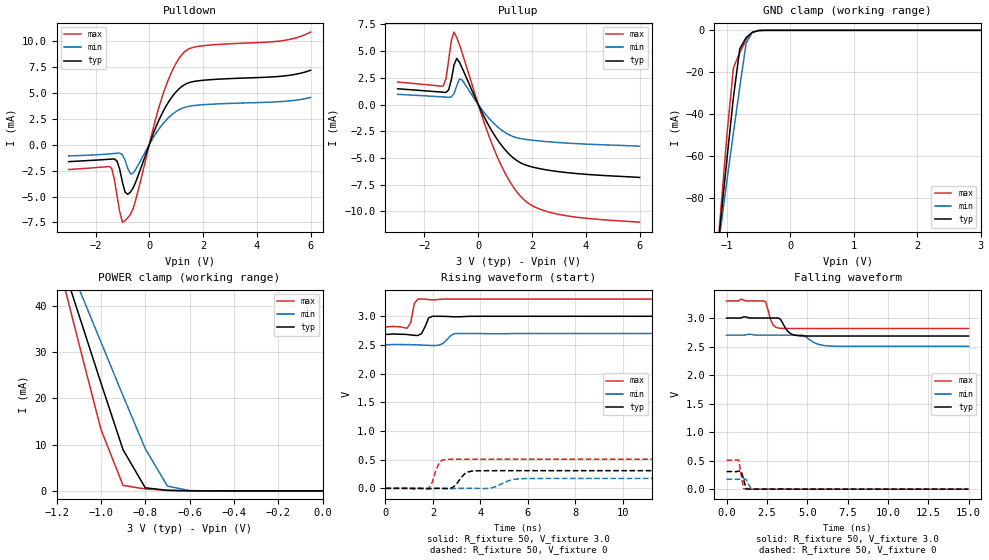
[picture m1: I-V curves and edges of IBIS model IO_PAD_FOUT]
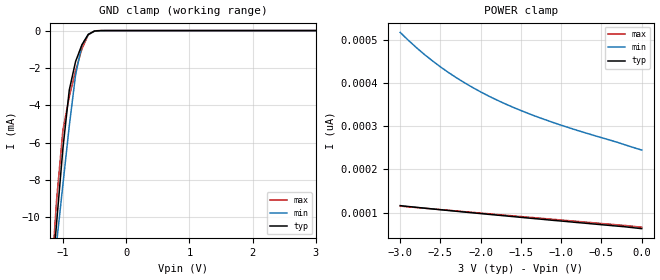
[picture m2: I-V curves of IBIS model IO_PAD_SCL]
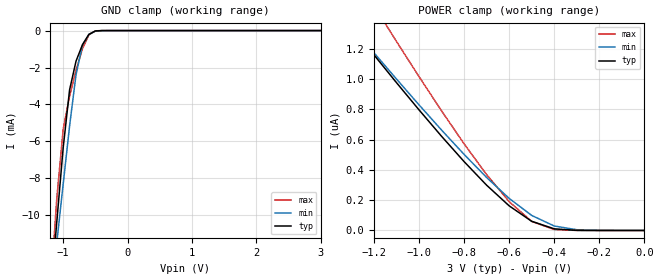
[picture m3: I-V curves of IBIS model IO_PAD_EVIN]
[IBIS Ver]   3.2
[Comment Char]   |_char
[File name]   rx8111ce_3v.ibs
[File Rev]   1.0
[Date]   2019/09/25 8:10:22
[Source]
[Notes]
[Disclaimer]
This information is for modeling purposes only, and is not guaranteed.
Property of SEIKO EPSON Corp.,
unauthorized reproduction and/or distribution is strictly prohibited.
[Copyright]
Copyright 2019, SEIKO EPSON Corp.
[Component]   T5462W0B
Si_location Pin
Timing_location Pin
[Manufacturer]   SEIKO EPSON Corp.
| RX-8111CE
[Package]
R_pkg   0.0m   0.0m   0.0m
L_pkg   0.0n   0.0n   0.0n
C_pkg   0.0p   0.0p   0.0p
[Pin] signal_name   model_name
1   VDD   POWER
2   VOUT   POWER
3   VBAT   POWER
4   FOUT   IO_PAD_FOUT
5   SCL   IO_PAD_SCL
6   EVIN   IO_PAD_EVIN
7   SDA   IO_PAD_SDA
8   VIO   POWER
9   GND   GND
10   /INT   IO_PAD_XINT
| Models and submodels in the file (5): IO_PAD_FOUT (3-state), IO_PAD_SCL (Input), IO_PAD_EVIN (Input), IO_PAD_SDA (I/O_open_drain), IO_PAD_XINT (Open_drain)
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[Model]   IO_PAD_FOUT
Model_type 3-state
Enable Active-High
Polarity Non-Inverting
Vmeas=1.50
C_comp   2.5p   2.0p   3.0p
[Temperature Range] 25   105   -40
[Voltage Range]   3.0   2.7   3.3
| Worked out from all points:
|   slope of the pulldown table from 0 to 0.45 V, typ, clamps not added: 158 ohm
|   slope of the pullup table from 0 to 0.45 V, typ, clamps not added: 202 ohm
|   GND clamp passes 1 mA (typ) near -0.60 V on its own axis
|   POWER clamp passes 1 mA (typ) near -0.80 V on its own axis
|   falling waveform, R_fixture 50, V_fixture 3.0: 20-80 % time 453ps typ, 696ps min, 319ps max; typ from 3 V to 2.69 V
|   falling waveform, R_fixture 50, V_fixture 0: 20-80 % time 184ps typ, 208ps min, 185ps max; typ from 0.309 V to 0 V
|   rising waveform, R_fixture 50, V_fixture 3.0: 20-80 % time 205ps typ, 279ps min, 132ps max; typ from 2.69 V to 3 V
|   rising waveform, R_fixture 50, V_fixture 0: 20-80 % time 365ps typ, 571ps min, 257ps max; typ from 0 V to 0.309 V
[Pullup]
-3V       1.471mA    952.6uA    2.104mA
-1.3V     1.147mA    709.8uA    1.738mA
-1.2V     1.13mA     694.5uA    2.414mA
-1.1V     1.366mA    679uA      4.16mA
-1V       2.339mA    705.4uA    6.008mA
-900mV    3.706mA    1.017mA    6.776mA
-800mV    4.313mA    1.748mA    6.271mA
-600mV    3.419mA    2.299mA    4.848mA
600mV     -2.854mA   -1.818mA   -4.245mA
1.6V      -5.487mA   -3.2mA     -8.66mA
2.9V      -6.251mA   -3.543mA   -10.23mA
6V        -6.823mA   -3.898mA   -11.01mA
[Pulldown]
-3V       -1.645mA   -1.105mA   -2.404mA
-1.4V     -1.401mA   -881.9uA   -2.281mA
-1.2V     -1.594mA   -838.2uA   -4.933mA
-1V       -3.61mA    -971.9uA   -7.472mA
-800mV    -4.793mA   -2.307mA   -7.046mA
-600mV    -4.172mA   -2.75mA    -6.158mA
500mV     3.112mA    1.977mA    4.757mA
900mV     4.773mA    3.003mA    7.349mA
1.3V      5.744mA    3.563mA    8.902mA
2V        6.182mA    3.832mA    9.508mA
5V        6.596mA    4.15mA     10.01mA
6V        7.149mA    4.527mA    10.82mA
[GND Clamp]
-3V       -666mA     -547.8mA   -822.2mA
-1.2V     -119.6mA   -117.1mA   -123.7mA
-1.1V     -89.89mA   -93.83mA   -85.8mA
-1V       -60.42mA   -70.86mA   -48.73mA
-900mV    -31.79mA   -48.51mA   -17.79mA
-800mV    -8.762mA   -26.99mA   -10.57mA
-700mV    -3.482mA   -6.087mA   -4.558mA
-600mV    -875.1uA   -938.3uA   -964.6uA
-500mV    -86.79uA   -136.7uA   -53.06uA
-400mV    -4.756uA   -14.79uA   -1.084uA
3V        37.81pA    65.05nA    23.86pA
[POWER Clamp]
-3V       323.7mA    269.5mA    395.6mA
-1.2V     53.06mA    55.67mA    50.96mA
-1.1V     38.19mA    43.92mA    32.03mA
-1V       23.39mA    32.21mA    13.33mA
-900mV    8.898mA    20.56mA    1.192mA
-800mV    679.8uA    9.149mA    426.2uA
-700mV    116.6uA    1.034mA    140.4uA
-600mV    22.63uA    76.12uA    22.74uA
0V        37.92pA    763.7pA    29.64pA
[Falling Waveform]
R_fixture=50
V_fixture=3.0
V_fixture_min=2.7
V_fixture_max=3.3
0s        3V         2.7V       3.3V
909.1ps   3.003V     2.699V     3.333V
2.424ns   3V         2.7V       3.286V
2.727ns   3V         2.7V       2.971V
2.879ns   3V         2.7V       2.883V
3.333ns   2.982V     2.7V       2.82V
3.788ns   2.77V      2.7V       2.817V
4.394ns   2.692V     2.7V       2.817V
6.364ns   2.685V     2.511V     2.816V
15ns      2.685V     2.505V     2.816V
[Falling Waveform]
R_fixture=50
V_fixture=0
V_fixture_min=0
V_fixture_max=0
0s        308.8mV    173.5mV    508.3mV
606.1ps   306.9mV    172.2mV    509.2mV
757.6ps   317.4mV    172.5mV    510.2mV
909.1ps   318.5mV    177.7mV    238.4mV
1.061ns   167.4mV    186mV      11.86mV
1.212ns   14.15mV    167.8mV    329.8uV
1.364ns   1.997mV    84.14mV    10.39uV
1.515ns   201.5uV    15.32mV    -15.29uV
1.818ns   11.09uV    1.012mV    -15.97uV
15ns      0V         0V         621.2nV
[Rising Waveform]
R_fixture=50
V_fixture=3.0
V_fixture_min=2.7
V_fixture_max=3.3
0s        2.685V     2.505V     2.816V
909.1ps   2.683V     2.506V     2.791V
1.061ns   2.675V     2.505V     2.887V
1.212ns   2.668V     2.505V     3.221V
1.364ns   2.666V     2.502V     3.299V
1.515ns   2.697V     2.499V     3.299V
1.818ns   2.971V     2.493V     3.291V
1.97ns    3V         2.491V     3.285V
3.03ns    2.991V     2.7V       3.3V
15ns      3V         2.7V       3.3V
[Rising Waveform]
R_fixture=50
V_fixture=0
V_fixture_min=0
V_fixture_max=0
0s        0V         0V         0V
1.818ns   -8.601mV   102.5uV    633.1uV
2.273ns   -361.6uV   -684.4uV   455.5mV
2.576ns   -2.263mV   -3.519mV   505.4mV
2.879ns   27.32mV    -4.664mV   507.4mV
3.333ns   253.3mV    3.654uV    508.1mV
3.788ns   305.3mV    -550.9uV   508.3mV
4.394ns   308.2mV    1.863mV    508.3mV
5.758ns   308.8mV    169.3mV    508.3mV
15ns      308.8mV    173.5mV    508.3mV
[Ramp]
R_load=50
dV/dt_r   1.853E-1/3.478E-10   1.041E-1/5.635E-10   3.050E-1/2.294E-10
dV/dt_f   1.891E-1/4.362E-10   1.172E-1/6.888E-10   2.901E-1/2.838E-10
|[End   IO_PAD_FOUT
[Model]   IO_PAD_SCL
Model_type Input
Enable Active-High
Polarity Non-Inverting
Vinh=2.64
Vinl=0.54
C_comp   2.5p   2.0p   3.0p
[Temperature Range] 25   105   -40
[Voltage Range]   3.0   2.7   3.3
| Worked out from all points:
|   GND clamp passes 1 mA (typ) near -0.73 V on its own axis
[GND Clamp]
-3V       -89.07mA   -73.01mA   -108.2mA
-1.2V     -14.34mA   -14.53mA   -14.15mA
-1.1V     -10.29mA   -11.38mA   -9.068mA
-1V       -6.299mA   -8.232mA   -5.325mA
-900mV    -3.19mA    -5.115mA   -3.551mA
-800mV    -1.656mA   -2.369mA   -2.158mA
-700mV    -763.9uA   -781.8uA   -983.1uA
-600mV    -207.7uA   -205.1uA   -228.8uA
-500mV    -21.87uA   -34.9uA    -13.49uA
-300mV    -47nA      -341.4nA   -3.543nA
3V        62.74pA    262.6pA    59.91pA
[POWER Clamp]
-3V       116.1pA    517.3pA    114.9pA
-2.9V     114.1pA    499.3pA    113.4pA
-2.7V     110.2pA    466.4pA    110.1pA
-2.5V     106.6pA    437.5pA    106.9pA
-2.2V     101.2pA    400.6pA    102pA
-1.9V     95.86pA    369.8pA    97.27pA
-1.6V     90.66pA    344.1pA    92.38pA
-1.2V     83.74pA    315.2pA    85.98pA
-800mV    76.94pA    290.4pA    79.61pA
0V        62.73pA    244.8pA    66.05pA
[Model]   IO_PAD_EVIN
Model_type Input
Enable Active-High
Polarity Non-Inverting
Vinh=2.64
Vinl=0.54
C_comp   2.5p   2.0p   3.0p
[Temperature Range] 25   105   -40
[Voltage Range]   3.0   2.7   3.3
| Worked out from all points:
|   GND clamp passes 1 mA (typ) near -0.73 V on its own axis
[GND Clamp]
-3V       -90.37mA   -74.11mA   -109.7mA
-1.2V     -14.51mA   -14.72mA   -14.31mA
-1.1V     -10.41mA   -11.52mA   -9.157mA
-1V       -6.36mA    -8.327mA   -5.354mA
-900mV    -3.209mA   -5.169mA   -3.552mA
-800mV    -1.657mA   -2.388mA   -2.158mA
-700mV    -764.4uA   -784.2uA   -983.6uA
-600mV    -208.1uA   -205.5uA   -229.1uA
-500mV    -22.03uA   -35.1uA    -13.63uA
-300mV    -50.61nA   -359nA     -4.103nA
3V        69.48pA    4.945nA    63.03pA
[POWER Clamp]
-3V       4.774uA    4.535uA    6.092uA
-1.3V     1.344uA    1.347uA    1.722uA
-1.2V     1.158uA    1.171uA    1.482uA
-1.1V     974.3nA    998.2nA    1.246uA
-900mV    620.8nA    661.9nA    788.3nA
-800mV    454nA      501.3nA    571.2nA
-700mV    298.4nA    349.2nA    367.9nA
-600mV    162.3nA    211.4nA    189.9nA
-500mV    60.44nA    99.19nA    59.87nA
-400mV    10.92nA    29.54nA    6.359nA
-300mV    859pA      4.944nA    249.5pA
0V        69.49pA    262pA      73.59pA
